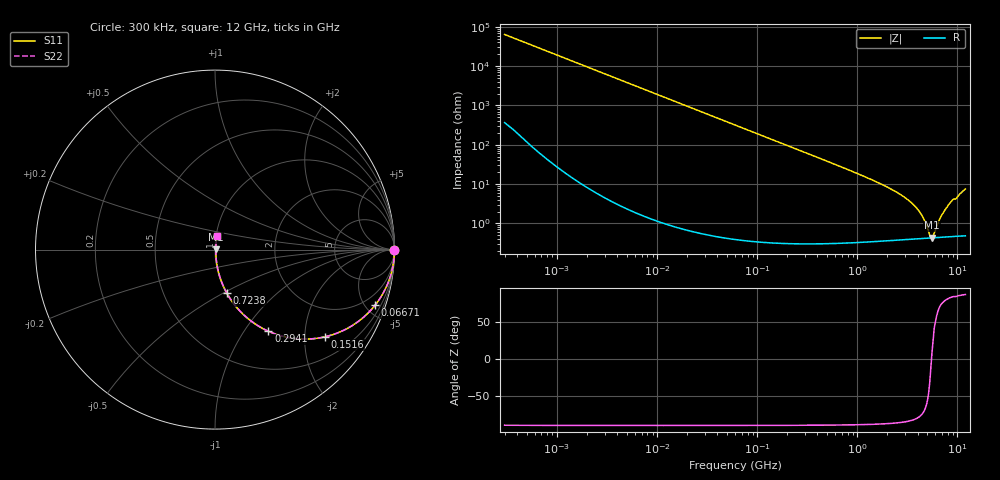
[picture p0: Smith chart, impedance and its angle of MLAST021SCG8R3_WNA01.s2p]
! MLAST021SCG8R3_WNA01  S-PARAMETER MODEL  ( General Type )
! Model Generated by TAIYO YUDEN Corporation (http://www.ty-top.com)
! Version 1.0
! TAIYO YUDEN Control No. 220901
! Copyright(c) 2022 TAIYO YUDEN CO.,LTD. All Rights Reserved.
! Product Description (link to TY-COMPAS)
! https://ds.yuden.co.jp/TYCOMPAS/or/detail?pn=MLAST021SCG8R3CWNA01&u=M
! Products Name : Multilayer Ceramic Capacitors
! Characteristics :
!  Capacitance : 8.3 pF , Rated Voltage : 25V , TCC : CG / C0G
!  Case Size : 0.25 x 0.125 / 0.0098 x 0.0049 [mm/inch] , Thickness : 0.125 / 0.0049 [mm/inch]
!  (Conditions: Temperature = 25 degC , DC Bias Current/Voltage = 0A / 0V)
! External Node Assignments :
!  1  o---| |---o  2
! GND o---------o GND
! Frequency Range : 0.3MHz  -  12000MHz  [ 401 STEP ]
# MHz S RI R 50
! Freq[MHz].  S11 Real  S11 Imag  S21 Real  S21 Imag  S12 Real  S12 Imag  S22 Real  S22 Imag
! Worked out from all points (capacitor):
!   401 points, 300 kHz to 12 GHz, reference 50 ohm
!   read as one part in series: C = 8.3 pF near 316.3 kHz
!   lowest |Z| = 433 mohm at 5.566 GHz (marker M1)
!   series resonance near 5.508 GHz, so ESL is about 100 pH
!   S11 on the Smith chart (normalised r, x): 300 kHz: open; 66.71 MHz: 1.01, -5.75; 151.6 MHz: 1.01, -2.53; 294.1 MHz: 1.01, -1.30; 723.8 MHz: 1.01, -0.52; 12 GHz: 1.01, +0.15
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0.3  1 -0.00156  1.14e-05 0.00156  1.14e-05 0.00156  1 -0.00156
1.769972  0.9999 -0.00923  9.36e-05 0.00923  9.36e-05 0.00923  0.9999 -0.00923
10.44266  0.997 -0.0543  0.00299 0.0543  0.00299 0.0543  0.997 -0.0543
27.10171  0.9803 -0.1385  0.0197 0.1385  0.0197 0.1385  0.9803 -0.1385
60  0.9105 -0.2848  0.0895 0.2848  0.0895 0.2848  0.9105 -0.2848
66.70707  0.8917 -0.3101  0.1083 0.3101  0.1083 0.3101  0.8917 -0.3101
99.25425  0.7882 -0.4077  0.2118 0.4077  0.2118 0.4077  0.7882 -0.4077
151.6462  0.6146 -0.4855  0.3854 0.4855  0.3854 0.4855  0.6146 -0.4855
294.0765  0.298 -0.4551  0.702 0.4551  0.702 0.4551  0.298 -0.4551
353.9943  0.2267 -0.4159  0.7733 0.4159  0.7733 0.4159  0.2267 -0.4159
723.8279  0.066 -0.2424  0.934 0.2424  0.934 0.2424  0.066 -0.2424
2088.533  0.00968 -0.0775  0.9903 0.0775  0.9903 0.0775  0.00968 -0.0775
3026.31  0.00577 -0.0437  0.9942 0.0437  0.9942 0.0437  0.00577 -0.0437
3841.137  0.00465 -0.0253  0.9953 0.0253  0.9953 0.0253  0.00465 -0.0253
4385.161  0.00435 -0.0157  0.9957 0.0157  0.9957 0.0157  0.00435 -0.0157
5278.635  0.00424 -0.00274  0.9958 0.00274  0.9958 0.00274  0.00424 -0.00274
5565.855  0.00427 0.000602  0.9957 -0.000602  0.9957 -0.000602  0.00427 0.000602
5868.704  0.00432 0.00382  0.9957 -0.00382  0.9957 -0.00382  0.00432 0.00382
6879.757  0.00463 0.0146  0.9954 -0.0146  0.9954 -0.0146  0.00463 0.0146
7854.144  0.00515 0.0252  0.9949 -0.0252  0.9949 -0.0252  0.00515 0.0252
8732.115  0.00588 0.0359  0.9941 -0.0359  0.9941 -0.0359  0.00588 0.0359
12000  0.0103 0.0737  0.9897 -0.0737  0.9897 -0.0737  0.0103 0.0737
